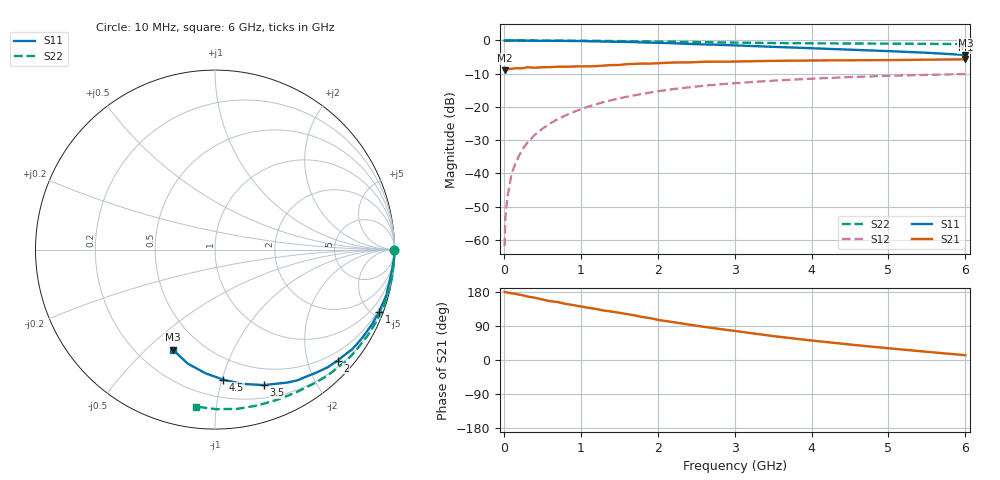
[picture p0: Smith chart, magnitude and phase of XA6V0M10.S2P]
! SIEMENS Discrete & RF Semiconductors
! BFY180
! Si NPN RF Bipolar Junction Transistor in MICRO-X
! VCE = 6 V  IC = 0.1 mA
! Common Emitter S-Parameters:  May  1997
# GHz  S  MA  R  50
!  f  S11  S21  S12  S22
! GHz  MAG  ANG  MAG  ANG  MAG  ANG  MAG  ANG
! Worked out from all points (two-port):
!   36 points, 10 MHz to 6 GHz, reference 50 ohm
!   highest |S21| = -5.70 dB at 6 GHz (marker M1); lowest = -9.0 dB at 10 MHz (marker M2)
!   |S21| within 3 dB of the highest: 16.77 MHz to end of sweep
!   lowest |S11| = -4.4 dB at 6 GHz (marker M3), VSWR 4.06, Z = 17.3 - j30.3 ohm
!   |S11| at or under -10 dB: nowhere
!   |S22| runs from -1.1 to 0.0 dB; largest |S21 - S12| = 0.4
!   S11 on the Smith chart (normalised r, x): 10 MHz: open; 1 GHz: 0.30, -5.43; 2 GHz: 0.31, -2.56; 3.5 GHz: 0.32, -1.37; 4.5 GHz: 0.33, -1.01; 6 GHz: 0.35, -0.61
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0.01  0.9952 -0.1  0.356 179.7  0.0008 89.9  0.9992 -0.1
0.02  0.9963 -0.4  0.373 178.9  0.0022 91.2  0.9999 -0.4
0.05  0.9941 -1.0  0.37 178.1  0.0046 86.1  0.9987 -0.9
0.1  0.9993 -2.1  0.375 176.1  0.0098 88.8  0.9977 -1.9
0.15  0.9981 -3.3  0.382 174.6  0.014 86.3  0.9999 -2.8
0.2  0.9961 -4.1  0.381 172.4  0.0186 85.9  0.9989 -3.8
0.25  0.994 -5.3  0.382 170.7  0.0236 85.7  0.9999 -4.7
0.3  0.9934 -6.3  0.394 167.8  0.0283 84.0  0.9978 -5.6
0.4  0.9897 -8.5  0.389 164.4  0.0377 82.5  0.9986 -7.5
0.5  0.989 -10.7  0.395 159.7  0.0468 80.4  0.9979 -9.4
0.7  0.989 -14.8  0.402 153.0  0.0654 76.1  0.9953 -13.2
1  0.9803 -20.8  0.408 141.3  0.0922 70.2  0.9902 -18.8
1.1  0.9718 -23.0  0.407 137.8  0.1009 68.5  0.9876 -20.5
1.3  0.9631 -27.5  0.418 130.5  0.1185 64.4  0.9836 -24.3
1.6  0.9489 -34.0  0.44 121.3  0.1422 58.7  0.9751 -29.9
2  0.9214 -42.2  0.454 106.0  0.1718 51.2  0.9639 -36.9
2.2  0.908 -46.2  0.466 99.9  0.1851 47.4  0.9584 -40.4
2.8  0.8605 -57.9  0.479 82.0  0.2183 37.1  0.9358 -50.1
3.5  0.8022 -70.2  0.493 63.1  0.2482 26.4  0.9148 -60.5
4.5  0.7264 -86.3  0.503 40.8  0.2808 12.7  0.8998 -74.9
5.5  0.6524 -103.6  0.514 21.6  0.3033 -0.2  0.889 -89.5
6  0.6044 -112.9  0.519 12.6  0.3118 -6.9  0.8811 -96.8
